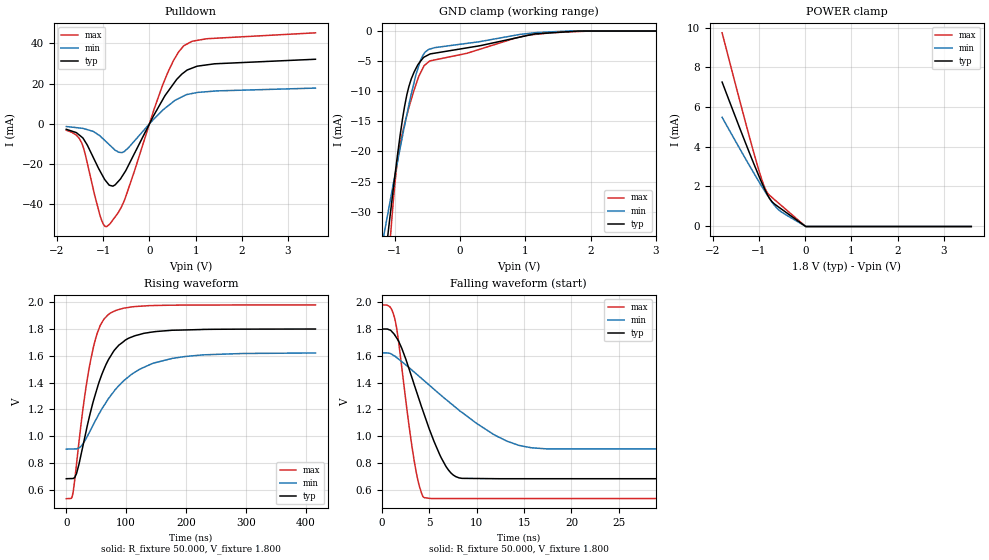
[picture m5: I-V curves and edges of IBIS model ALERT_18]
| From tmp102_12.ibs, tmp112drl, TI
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|   ALERT_18   1.8V digital open-drain Model
[Model] ALERT_18
Model_type   Open_drain
| Signals   ALERT(3)
Polarity   Non-Inverting
Enable   Active-Low
Vmeas = 0.9
Vref = 0.9
Cref = 15pF
Rref = 50
|   typ   min   max
|   (nom PVT)   (Fast PVT)   (slow PVT)
|   output low
|C_comp   1.5662960e-10  7.6417880e-11  1.2725910e-10
| Where   nom PVT is  Nominal Process, 1.8V, -40C
|   Fast PVT is Strong Process, 1.98V, 125C
|   Slow PVT is Weak Process, 1.62V, 27C
|   output high
C_comp   1.3417690e-12  1.2431060e-12  1.5132630e-12
| Where   nom PVT is  Nominal Process, 1.5V, 27C
|   Fast PVT is Strong Process, 1.6V, -40C
|   Slow PVT is Weak Process, 1.4V, 125C
[Voltage Range]   1.8   1.62   1.98
[Temperature Range]   27   125   -40
|Ambient Temperature   27   125   -40
[Pullup Reference]   1.8   1.62   1.98
[Pulldown Reference]   0   0   0
[Power Clamp Reference]   1.8   1.62   1.98
[GND Clamp Reference]   0   0   0
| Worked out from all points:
|   slope of the pulldown table from 0 to 0.27 V, typ, clamps not added: 23.8 ohm
|   POWER clamp passes 1 mA (typ) near -0.60 V on its own axis
|   falling waveform, R_fixture 50.000, V_fixture 1.800: 20-80 % time 3.31ns typ, 7.61ns min, 1.61ns max; typ from 1.8 V to 0.681 V
|   rising waveform, R_fixture 50.000, V_fixture 1.800: 20-80 % time 44.4ns typ, 74ns min, 29ns max; typ from 0.681 V to 1.8 V
[Pulldown]
|   Voltage   I(typ)   I(min)   I(max)
-1.8V     -2.736mA   -1.352mA   -3.231mA
-1.464V   -6.595mA   -2.199mA   -9.594mA
-1.075V   -23.24mA   -5.932mA   -45.1mA
-993.4mV  -26.65mA   -7.673mA   -50.07mA
-925.5mV  -28.92mA   -9.144mA   -51.05mA
-789.4mV  -30.95mA   -12.09mA   -47.67mA
-553.6mV  -24.76mA   -13.92mA   -38.64mA
282.8mV   11.81mA    6.634mA    19.02mA
525.1mV   19.97mA    11.11mA    31.57mA
737.1mV   25.3mA     13.77mA    38.58mA
1.412V    29.79mA    16.24mA    42.45mA
3.595V    32.04mA    17.72mA    45.17mA
[GND Clamp]
|   Voltage   I(typ)   I(min)   I(max)
-1.8V     -102.9mA   -72.35mA   -157.3mA
-1.193V   -42.27mA   -35.42mA   -53.62mA
-1.131V   -36.28mA   -31.74mA   -43.72mA
-1.092V   -32.56mA   -29.46mA   -37.9mA
-1.075V   -30.98mA   -28.45mA   -35.34mA
-1.03V    -26.87mA   -25.81mA   -29.19mA
-943.4mV  -19.35mA   -20.9mA    -20.33mA
-811.5mV  -10.41mA   -13.71mA   -13.85mA
-611.5mV  -5.098mA   -5.032mA   -7.074mA
-476.9mV  -3.907mA   -3.033mA   -5.08mA
1.048V    -704.9uA   -401.4uA   -674.1uA
3.595V    0A         0A         0A
[POWER Clamp]
|   Voltage   I(typ)   I(min)   I(max)
-1.8V     7.252mA    5.479mA    9.733mA
-1.414V   4.908mA    3.884mA    6.281mA
-1.157V   3.39mA     2.845mA    4.054mA
-982.5mV  2.408mA    2.162mA    2.649mA
-869.8mV  1.824mA    1.737mA    1.899mA
-819.6mV  1.589mA    1.555mA    1.679mA
-730.1mV  1.259mA    1.245mA    1.466mA
-636.4mV  1.063mA    962.1uA    1.277mA
-561.3mV  935.4uA    789.6uA    1.126mA
10.99mV   -18.31uA   -14.99uA   -22.06uA
3.595V    -18.31uA   -14.99uA   -22.06uA
[Ramp]
R_load = 50
|   typ   min   max
dV/dt_r   0.67123/4.4312e-008   0.424628/7.37221e-008   0.86876/2.89414e-008
dV/dt_f   0.67123/3.30337e-009  0.424628/7.56536e-009   0.86876/1.60515e-009
[Falling Waveform]
R_fixture = 50.000
V_fixture = 1.800
V_fixture_min = 1.620
V_fixture_max = 1.980
C_fixture = 0.000
|  time   V(typ)   V(min)   V(max)
0s        1.8V       1.621V     1.98V
1.376ns   1.755V     1.597V     1.877V
3.681ns   1.329V     1.462V     713.7mV
4.336ns   1.19V      1.422V     549mV
5.154ns   1.026V     1.372V     533.4mV
6.759ns   774.5mV    1.274V     533.4mV
7.813ns   696.8mV    1.213V     533.4mV
13.19ns   681.3mV    962.4mV    533.3mV
17.4ns    681.3mV    904.2mV    533.3mV
416.6ns   681.3mV    902.6mV    532.1mV
[Rising Waveform]
R_fixture = 50.000
V_fixture = 1.800
V_fixture_min = 1.620
V_fixture_max = 1.980
C_fixture = 0.000
|  time   V(typ)   V(min)   V(max)
0s        681.3mV    902.6mV    532.1mV
11.21ns   683.1mV    903.7mV    574.9mV
17.4ns    724.6mV    904.7mV    802.9mV
30.19ns   975.1mV    958.8mV    1.279V
45.56ns   1.266V     1.089V     1.668V
56.52ns   1.425V     1.179V     1.824V
70.47ns   1.571V     1.279V     1.908V
104.7ns   1.732V     1.445V     1.962V
177.4ns   1.791V     1.581V     1.978V
416.6ns   1.8V       1.621V     1.98V
